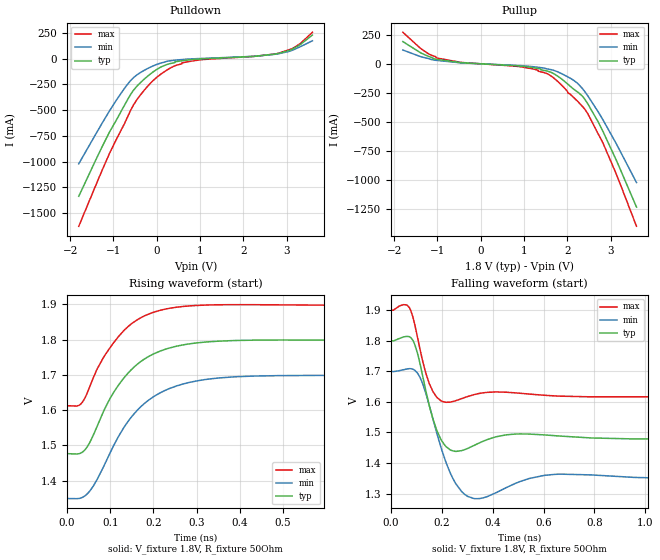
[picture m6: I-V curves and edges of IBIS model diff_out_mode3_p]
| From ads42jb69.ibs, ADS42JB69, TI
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|   diff_out_mode3 Model
[Model]   diff_out_mode3_p
Model_type   Output
Polarity   Non-Inverting
Vmeas = 1.6481
Vref = 1.8
Cref = 0.5pF
Rref = 50
|   typ   min   max
|   (nom PVT)   (fast PVT)   (slow PVT)
C_comp   2.726e-12   2.331e-12   2.910e-12
[Model spec]
|subparameter   typ   min   max
Vmeas   1.6481   1.545   1.7588
| Where nom  PVT is Nominal Process, 1.8V, 25C
|   Fast PVT is Strong Process,  1.9V, -40C
|   Slow PVT is Weak Process,   1.7V, 125C
[Voltage Range]   1.8   1.7   1.9
[Temperature Range]   25   125   -40
[Pullup Reference]   1.8   1.7   1.9
[Pulldown Reference]   0   0   0
[Power Clamp Reference]   1.8   1.7   1.9
[GND Clamp Reference]   0   0   0
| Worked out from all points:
|   slope of the pulldown table from 0 to 0.27 V, typ, clamps not added: 5.14 ohm
|   slope of the pullup table from 0 to 0.27 V, typ, clamps not added: 49.1 ohm
|   falling waveform, V_fixture 1.8V, R_fixture 50Ohm: 20-80 % time 54.3ps typ, 72.7ps min, 50.2ps max; typ from 1.8 V to 1.48 V
|   rising waveform, V_fixture 1.8V, R_fixture 50Ohm: 20-80 % time 101ps typ, 113ps min, 91.2ps max; typ from 1.48 V to 1.8 V
[Pulldown]
|   Voltage   I(typ)   I(min)   I(max)
-1.8V     -1.337A    -1.021A    -1.629A
-1.094V   -716.9mA   -511.2mA   -925.4mA
-621mV    -361.5mA   -222.3mA   -519.6mA
-538.2mV  -308.5mA   -185.7mA   -451.8mA
-373.1mV  -232.4mA   -134.5mA   -351.9mA
-700uV    -105.6mA   -56.64mA   -182.3mA
316.5mV   -47.47mA   -20.42mA   -90.78mA
621mV     -18.51mA   -7.368mA   -37.78mA
2.817V    50.52mA    47.87mA    52.44mA
3.133V    91.34mA    81.3mA     97.45mA
3.328V    140.2mA    118.2mA    150.4mA
3.598V    229.5mA    173.6mA    256.3mA
[Pullup]
|   Voltage   I(typ)   I(min)   I(max)
-1.8V     191.5mA    118.9mA    271.6mA
-1.368V   90.53mA    59.59mA    126.1mA
-1.036V   39.14mA    29.93mA    51.34mA
1.005V    -22.9mA    -18.07mA   -31.06mA
1.324V    -40.25mA   -29.94mA   -54.89mA
1.694V    -86.61mA   -57.37mA   -124.8mA
2.154V    -220.5mA   -144.3mA   -293mA
2.338V    -275.2mA   -208.8mA   -362.8mA
2.474V    -345.7mA   -276.2mA   -430.8mA
2.829V    -587.8mA   -486.8mA   -688mA
3.167V    -860.7mA   -714.3mA   -983.2mA
3.598V    -1.235A    -1.024A    -1.401A
[Ramp]
R_load = 50
|   typ   min   max
dV/dt_r   0.0914551/4.91666e-11  0.120014/6.51689e-11   0.0741903/4.16294e-11
dV/dt_f   0.192481/5.42264e-11   0.209677/7.25395e-11   0.169614/4.87399e-11
[Falling Waveform]
V_fixture = 1.8V
V_fixture_min = 1.7V
V_fixture_max = 1.9V
R_fixture = 50Ohm
C_fixture = 0F
|   Time   V(typ)   V(min)   V(max)
0s        1.799V     1.699V     1.899V
61ps      1.814V     1.707V     1.917V
86.5ps    1.799V     1.706V     1.874V
138ps     1.631V     1.623V     1.69V
180.5ps   1.505V     1.495V     1.614V
251ps     1.438V     1.337V     1.603V
326.5ps   1.458V     1.284V     1.624V
455ps     1.492V     1.32V      1.631V
664.5ps   1.488V     1.364V     1.619V
1.999ns   1.478V     1.35V      1.613V
[Rising Waveform]
V_fixture = 1.8V
V_fixture_min = 1.7V
V_fixture_max = 1.9V
R_fixture = 50Ohm
C_fixture = 0F
|   Time   V(typ)   V(min)   V(max)
0s        1.477V     1.349V     1.613V
31.5ps    1.478V     1.35V      1.617V
53ps      1.509V     1.371V     1.668V
87ps      1.603V     1.446V     1.755V
109.5ps   1.653V     1.503V     1.794V
143ps     1.707V     1.571V     1.839V
193.5ps   1.755V     1.632V     1.875V
253.5ps   1.781V     1.669V     1.892V
432.5ps   1.799V     1.697V     1.899V
934.5ps   1.798V     1.698V     1.898V
